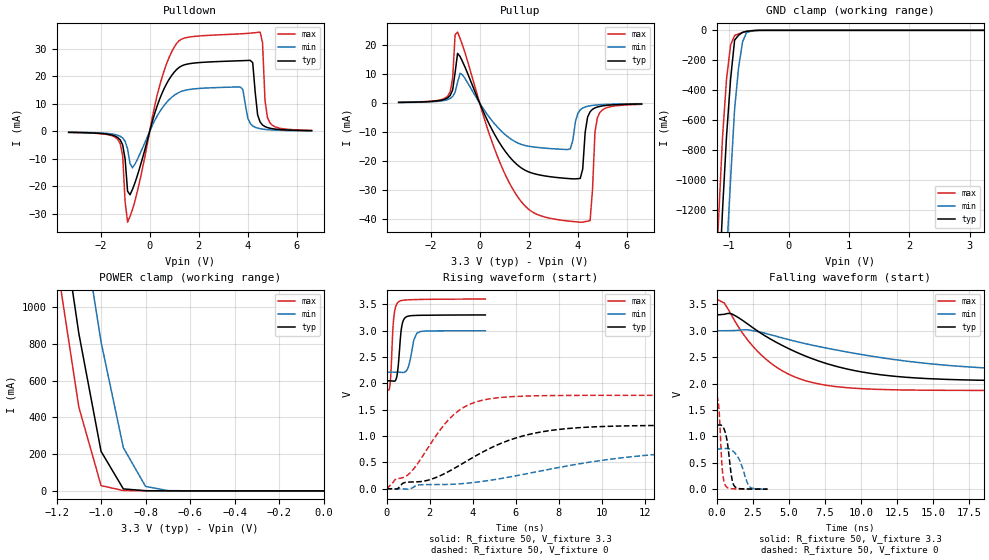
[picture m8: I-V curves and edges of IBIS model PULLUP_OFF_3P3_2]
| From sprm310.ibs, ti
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|   Model Cell PULLUP_OFF_3P3
|PULLUP_OFF_3P3
[Model]   PULLUP_OFF_3P3_2
Model_type   I/O
Polarity   Non-Inverting
Enable   Active-Low
Vinl =  0.8v
Vinh =  2v
Cref =  15.0000pF
Rref =  100.0000M
Vref =  0V
Vmeas =  1.65
C_comp   2.2653p   1.9017p   2.9162p
[Model Spec]
Vinl   0.8v   0.8v   0.8v
Vinh   2v   2v   2v
[Temperature Range]   25   125   -40
[Voltage Range]   3.3   3   3.6
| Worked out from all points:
|   slope of the pulldown table from 0 to 0.495 V, typ, clamps not added: 36.1 ohm
|   slope of the pullup table from 0 to 0.495 V, typ, clamps not added: 54.7 ohm
|   GND clamp passes 1 mA (typ) near -0.56 V on its own axis
|   POWER clamp passes 1 mA (typ) near -0.79 V on its own axis
|   rising waveform, R_fixture 50, V_fixture 3.3: 20-80 % time 160ps typ, 230ps min, 134ps max; typ from 2.05 V to 3.3 V
|   rising waveform, R_fixture 50, V_fixture 0: 20-80 % time 3.57ns typ, 6.71ns min, 1.95ns max; typ from 0 V to 1.21 V
|   falling waveform, R_fixture 50, V_fixture 3.3: 20-80 % time 6.15ns typ, 10.1ns min, 3.6ns max; typ from 3.3 V to 2.05 V
|   falling waveform, R_fixture 50, V_fixture 0: 20-80 % time 341ps typ, 609ps min, 211ps max; typ from 1.21 V to 0.002 V
[POWER_clamp]
|   voltage   I(typ)   I(min)   I(max)
-3.3V     22.02A     22.67A     21.68A
-1.2V     1.685A     2.433A     1.254A
-1.167V   1.409A     2.149A     988.2mA
-1.133V   1.134A     1.865A     722.7mA
-1.1V     858.4mA    1.581A     457.2mA
-1.033V   429.7mA    1.068A     171.8mA
-1V       215.3mA    810.7mA    29.13mA
-900mV    11.02mA    235.7mA    2.078mA
-800mV    1.044mA    24.39mA    1.114mA
-700mV    433.7uA    1.869mA    539.5uA
-11.55fV  39.74pA    5.746nA    492.9fA
[Pulldown]
|   voltage   I(typ)   I(min)   I(max)
-3.3V     -316.2uA   -252uA     -342.5uA
-1.3V     -2.194mA   -1.367mA   -2.881mA
-1.1V     -4.864mA   -2.357mA   -8.68mA
-900mV    -21.69mA   -6.326mA   -32.98mA
-700mV    -21.05mA   -13.22mA   -28.38mA
1.1V      22.53mA    13.73mA    32.03mA
3.7V      25.72mA    16.14mA    35.5mA
4.1V      25.85mA    2.912mA    35.75mA
4.5V      3.467mA    1.014mA    36.14mA
4.7V      1.789mA    754.6uA    11.41mA
4.9V      1.189mA    599.4uA    3.155mA
6.6V      300.9uA    215.3uA    389.5uA
[Pullup]
|   voltage   I(typ)   I(min)   I(max)
-3.3V     241.9uA    204.6uA    268.8uA
-1.3V     1.834mA    1.218mA    2.447mA
-1.1V     4.579mA    2.274mA    8.648mA
-900mV    17.22mA    7.132mA    24.6mA
500mV     -9.137mA   -6.075mA   -13.34mA
1.5V      -21.13mA   -13.59mA   -31.84mA
3.7V      -26.2mA    -15.78mA   -40.94mA
4.1V      -26.07mA   -2.353mA   -41.26mA
4.5V      -3.012mA   -927.6uA   -40.7mA
4.7V      -1.665mA   -705uA     -9.946mA
4.9V      -1.139mA   -567.3uA   -3.253mA
6.6V      -301.5uA   -210.8uA   -437.2uA
[GND_clamp]
|   voltage   I(typ)   I(min)   I(max)
-3.3V     -22.43A    -23.21A    -22A
-1.233V   -2.355A    -3.229A    -1.845A
-1.167V   -1.767A    -2.634A    -1.265A
-1.1V     -1.196A    -2.049A    -708.9mA
-1.033V   -702mA     -1.501A    -322.6mA
-966.7mV  -325.1mA   -993.1mA   -97.67mA
-900mV    -65.05mA   -524.7mA   -34.13mA
-833.3mV  -32.46mA   -245.5mA   -23.5mA
-766.7mV  -12.99mA   -75.07mA   -14.37mA
-700mV    -6.634mA   -13.45mA   -6.743mA
-433.3mV  -69.28uA   -246.8uA   -22.58uA
3.233V    38.18pA    520.5nA    433.7fA
[Ramp]
| variable   typ   min   max
dV/dt_f  0.7695933/6.177126n   0.4842534/10.20328n   1.063263/3.616703n
dV/dt_r  0.7297848/3.59705n   0.4619729/6.831216n   1.070183/1.956169n
R_load = 50
[Rising Waveform]
R_fixture = 50
V_fixture = 3.3
V_fixture_min = 3
V_fixture_max = 3.6
|   time   V(typ)   V(min)   V(max)
0s        2.047V     2.212V     1.87V
152ps     2.047V     2.212V     1.94V
200ps     2.047V     2.213V     2.172V
328ps     2.042V     2.213V     3.207V
456ps     2.094V     2.212V     3.488V
544ps     2.334V     2.211V     3.541V
688ps     3.03V      2.208V     3.57V
920ps     3.261V     2.237V     3.582V
1.408ns   3.289V     2.951V     3.59V
4.592ns   3.297V     2.997V     3.599V
[Rising Waveform]
R_fixture = 50
V_fixture = 0
V_fixture_min = 0
V_fixture_max = 0
|   time   V(typ)   V(min)   V(max)
0s        59.65pV    15.83nV    1.383pV
392ps     -4.362mV   106.6uV    172mV
1.112ns   128.5mV    58.99uV    309.1mV
2.064ns   179.6mV    79.74mV    864.4mV
3.144ns   386.5mV    87.7mV     1.414V
4.712ns   748.8mV    155mV      1.701V
6.808ns   1.049V     309.3mV    1.763V
9.496ns   1.172V     508.8mV    1.772V
15.15ns   1.205V     711.5mV    1.773V
26.5ns    1.207V     759.2mV    1.773V
[Falling Waveform]
R_fixture = 50
V_fixture = 3.3
V_fixture_min = 3
V_fixture_max = 3.6
|   time   V(typ)   V(min)   V(max)
0s        3.3V       3V         3.6V
536ps     3.311V     3V         3.525V
1.056ns   3.32V      3.003V     3.287V
2.272ns   3.105V     3.015V     2.785V
3.832ns   2.828V     2.918V     2.371V
5.496ns   2.598V     2.797V     2.117V
7.672ns   2.374V     2.669V     1.964V
12.1ns    2.144V     2.462V     1.883V
19.13ns   2.059V     2.288V     1.87V
40.23ns   2.047V     2.215V     1.87V
[Falling Waveform]
R_fixture = 50
V_fixture = 0
V_fixture_min = 0
V_fixture_max = 0
|   time   V(typ)   V(min)   V(max)
0s        1.207V     762.2mV    1.773V
176ps     1.216V     762.7mV    1.493V
344ps     1.209V     766.1mV    592.2mV
424ps     1.188V     767.7mV    301.5mV
616ps     1.062V     770.3mV    72.13mV
776ps     833.8mV    767.4mV    25.36mV
1.032ns   252.4mV    741.5mV    9.872mV
1.24ns    57.32mV    694.8mV    6.785mV
2.312ns   3.629mV    41.04mV    1.554mV
3.528ns   1.609mV    3.02mV     679.5uV
